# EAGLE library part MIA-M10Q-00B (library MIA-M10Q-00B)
u-blox M10 GNSS System-in-Package ROM, TCXO, SAW, LNA, 1.8/3V 4.5 x 4.5 mm, S-LGA 53, Source: Datasheet
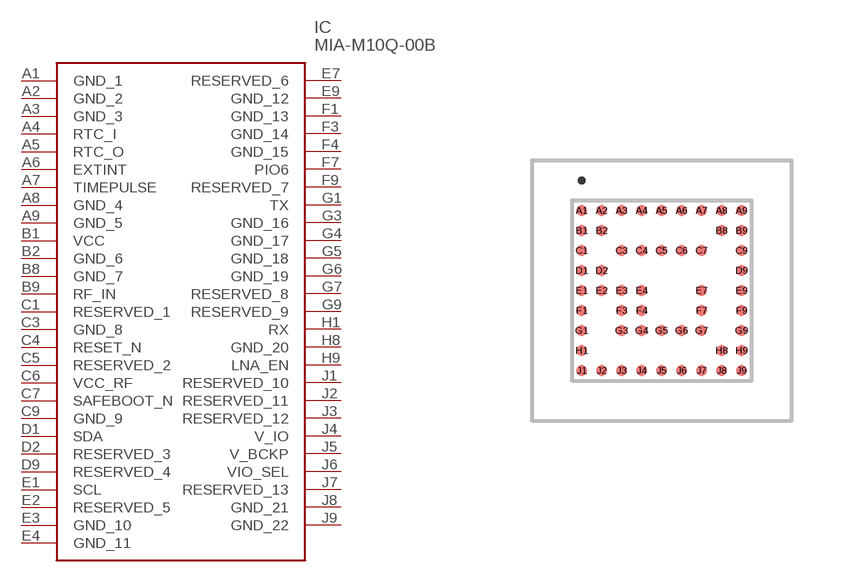
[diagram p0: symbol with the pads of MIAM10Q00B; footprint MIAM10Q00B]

Designator prefix IC

## MIA-M10Q-00B (Description: u-blox M10 GNSS System-in-Package ROM, TCXO, SAW, LNA, 1.8/3V 4.5 x 4.5 mm, S-LGA 53,; Height: 1.045mm; Manufacturer_Name: u-blox; Manufacturer_Part_Number: MIA-M10Q-00B; Mouser_Part_Number: 377-MIA-M10Q-00B; Mouser_Price-Stock: https://www.mouser.co.uk/ProductDetail/u-blox/MIA-M10Q-00B?qs=4ASt3YYao0VBtAexfwtW5Q%3D%3D)  [MIAM10Q00B]
A1  GND_1
A2  GND_2
A3  GND_3
A4  RTC_I
A5  RTC_O
A6  EXTINT
A7  TIMEPULSE
A8  GND_4
A9  GND_5
B1  VCC
B2  GND_6
B8  GND_7
B9  RF_IN
C1  RESERVED_1
C3  GND_8
C4  RESET_N
C5  RESERVED_2
C6  VCC_RF
C7  SAFEBOOT_N
C9  GND_9
D1  SDA
D2  RESERVED_3
D9  RESERVED_4
E1  SCL
E2  RESERVED_5
E3  GND_10
E4  GND_11
E7  RESERVED_6
E9  GND_12
F1  GND_13
F3  GND_14
F4  GND_15
F7  PIO6
F9  RESERVED_7
G1  TX
G3  GND_16
G4  GND_17
G5  GND_18
G6  GND_19
G7  RESERVED_8
G9  RESERVED_9
H1  RX
H8  GND_20
H9  LNA_EN
J1  RESERVED_10
J2  RESERVED_11
J3  RESERVED_12
J4  V_IO
J5  V_BCKP
J6  VIO_SEL
J7  RESERVED_13
J8  GND_21
J9  GND_22

## Footprint MIAM10Q00B (pad centres in mm)
MIA-M10Q-00B-1
smd 0.27 x 0.27: A1 -2,2; A2 -1.5,2; A3 -1,2; A4 -0.5,2; A5 0,2; A6 0.5,2; A7 1,2; A8 1.5,2; A9 2,2; B1 -2,1.5; B2 -1.5,1.5; B8 1.5,1.5; B9 2,1.5; C1 -2,1; C3 -1,1; C4 -0.5,1; C5 0,1; C6 0.5,1; C7 1,1; C9 2,1; D1 -2,0.5; D2 -1.5,0.5; D9 2,0.5; E1 -2,0; E2 -1.5,0; E3 -1,0; E4 -0.5,0; E7 1,0; E9 2,0; F1 -2,-0.5; F3 -1,-0.5; F4 -0.5,-0.5; F7 1,-0.5; F9 2,-0.5; G1 -2,-1; G3 -1,-1; G4 -0.5,-1; G5 0,-1; G6 0.5,-1; G7 1,-1; G9 2,-1; H1 -2,-1.5; H8 1.5,-1.5; H9 2,-1.5; J1 -2,-2; J2 -1.5,-2; J3 -1,-2; J4 -0.5,-2; J5 0,-2; J6 0.5,-2; J7 1,-2; J8 1.5,-2; J9 2,-2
